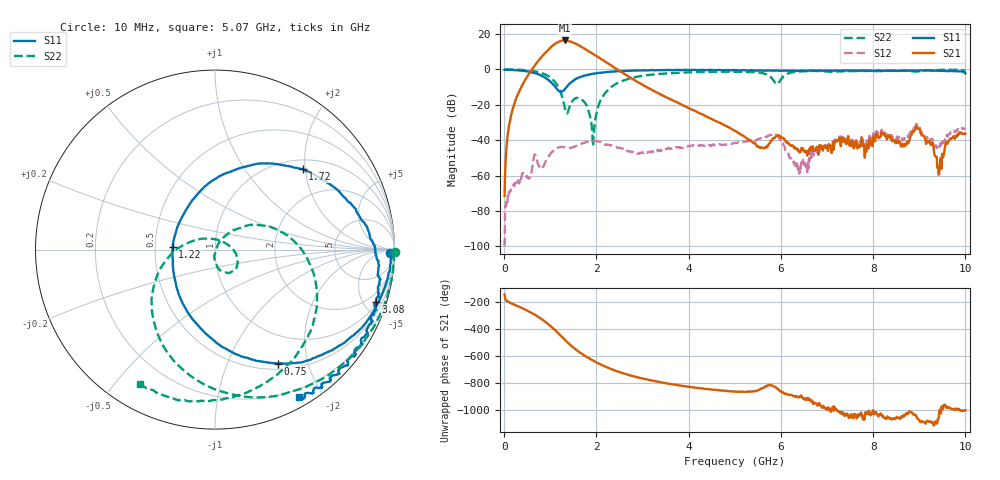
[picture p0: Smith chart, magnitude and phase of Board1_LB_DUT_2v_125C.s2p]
! Created Tue May 27 17:12:34 2025
# hz S ma R 50
! 2 Port Network Data from SP1.SP block
! freq  magS11  angS11  magS21  angS21  magS12  angS12  magS22  angS22
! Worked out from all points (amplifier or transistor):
!   1000 points, 10 MHz to 10 GHz, reference 50 ohm
!   highest |S21| = 16.4 dB at 1.31 GHz (marker M1)
!   |S21| within 3 dB of that: 1.048 GHz to 1.635 GHz (587 MHz wide, 43.7 % of centre)
!   unconditionally stable (mu >= 1): 15.59 MHz to 47.83 MHz; 51.37 MHz to end of sweep
!   at 1.67 GHz: K = 8.64, MAG = 15.1 dB, |S12| = -42.1 dB
!   at 5.01 GHz: K = 54.25, MAG = -17.0 dB, |S12| = -41.5 dB
!   at 10 GHz: K = 95.21, MAG = -24.2 dB, |S12| = -33.7 dB
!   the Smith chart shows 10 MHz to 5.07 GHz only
!   S11 on the Smith chart (normalised r, x): 10 MHz: 54, -44; 750 MHz: 0.57, -1.54; 1.22 GHz: 0.62, +0.02; 1.72 GHz: 1.21, +1.94; 3.08 GHz: 1.19, -6.08; 5.07 GHz: 0.11, -1.71
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1e7  0.9778 -1.0  0.0002681 -141.8  1.015e-05 92.4  1.003 -0.9
2e8  0.9657 -13.7  0.08871 146.3  0.0005556 78.0  0.9924 -17.8
7.5e8  0.7261 -61.0  1.807 49.2  0.001865 64.7  0.8368 -78.4
9e8  0.577 -80.9  3.05 13.2  0.002533 108.8  0.7128 -101.5
1.04e9  0.406 -108.2  4.582 -26.4  0.004663 99.4  0.5391 -128.4
1.13e9  0.2988 -136.1  5.591 -55.1  0.005888 85.3  0.3944 -149.5
1.22e9  0.2369 176.8  6.326 -85.7  0.006423 70.6  0.2329 -176.1
1.31e9  0.2718 127.0  6.609 -116.7  0.006329 60.5  0.09086 137.5
1.47e9  0.4515 77.1  5.948 -167.6  0.006192 57.2  0.1228 -14.2
1.68e9  0.6342 46.1  4.332 137.5  0.00802 49.1  0.1432 -63.5
1.72e9  0.6631 42.6  4.045 128.5  0.008318 46.3  0.1267 -71.3
1.93e9  0.7594 26.0  2.763 85.6  0.009476 25.9  0.006819 -2.2
2.12e9  0.8156 15.4  1.916 52.7  0.008619 5.0  0.156 45.4
2.5e9  0.8927 -1.0  0.9176 0.3  0.006169 -6.2  0.4411 6.4
3.08e9  0.9414 -18.0  0.3216 -53.8  0.004495 8.1  0.6846 -37.1
3.34e9  0.9568 -24.4  0.2135 -71.9  0.005338 9.1  0.7418 -52.4
5.01e9  0.9666 -59.3  0.01838 -144.8  0.008437 -10.3  0.8603 -116.8
5.07e9  0.9457 -60.3  0.01623 -146.3  0.008668 -10.9  0.8547 -119.1
6.67e9  0.9292 -90.0  0.005695 147.0  0.003732 139.9  0.9076 -150.6
8.34e9  0.9126 -134.8  0.01396 20.6  0.01602 32.1  0.9227 172.7
9.43e9  0.9142 -166.1  0.001094 63.0  0.006338 59.8  0.9656 168.6
1e10  0.7751 176.2  0.01518 76.3  0.02074 67.6  0.9225 168.3
